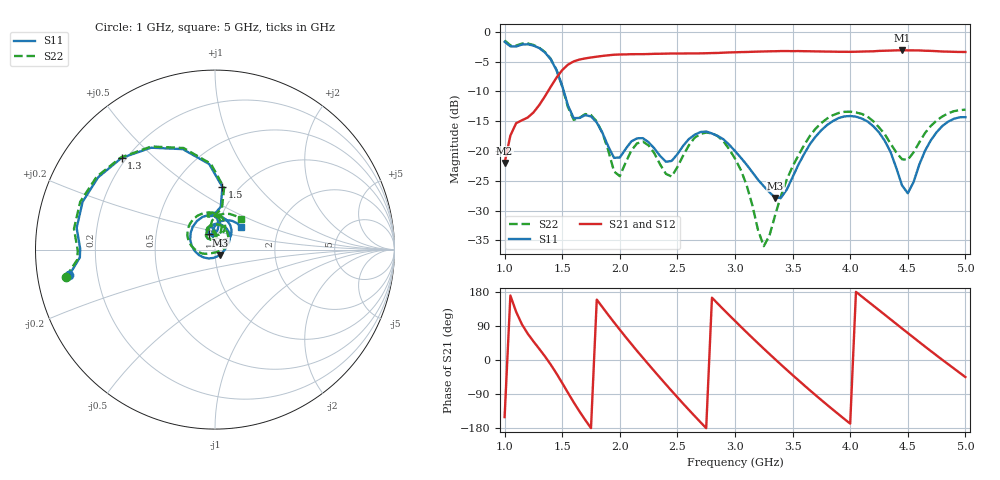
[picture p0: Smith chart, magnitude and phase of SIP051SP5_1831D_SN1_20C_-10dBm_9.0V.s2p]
# GHz  S  dB  R  50
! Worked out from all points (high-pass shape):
!   81 points, 1 GHz to 5 GHz, reference 50 ohm
!   highest |S21| = -3.12 dB at 4.45 GHz (marker M1); lowest = -22.0 dB at 1 GHz (marker M2)
!   |S21| within 3 dB of the highest: 1.518 GHz to end of sweep
!   lowest |S11| = -27.9 dB at 3.35 GHz (marker M3), VSWR 1.08, Z = 52.7 - j3.11 ohm
!   |S11| at or under -10 dB: 1.514 GHz to end of sweep
!   |S22| runs from -36.0 to -1.5 dB; largest |S21 - S12| = 0.002
!   S11 on the Smith chart (normalised r, x): 1 GHz: 0.10, -0.09; 1.3 GHz: 0.18, +0.40; 1.5 GHz: 0.84, +0.67; 2.5 GHz: 0.92, +0.16; 5 GHz: 1.29, +0.34
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1  -1.69 -170.2  -22.02 -150.6  -22.03 -150.5  -1.47 -169.7
1.1  -2.48 179.6  -15.35 127.2  -15.34 127.2  -2.33 -179.7
1.3  -2.74 135.6  -12.32 29.7  -12.35 29.6  -2.68 135.6
1.5  -9.10 83.2  -6.44 -60.7  -6.42 -60.8  -9.19 81.6
1.6  -14.50 93.5  -4.98 -111.8  -4.97 -111.8  -14.79 92.9
1.7  -14.01 100.4  -4.48 -158.3  -4.49 -158.3  -13.81 100.6
1.85  -17.00 81.3  -4.06 139.0  -4.05 139.0  -17.02 73.8
2  -21.11 109.3  -3.82 79.9  -3.82 80.0  -24.23 110.7
2.2  -17.86 99.9  -3.77 6.0  -3.77 5.9  -18.44 103.2
2.35  -20.85 90.9  -3.70 -47.0  -3.71 -47.0  -22.27 87.5
2.5  -20.55 111.7  -3.66 -98.3  -3.66 -98.3  -22.70 123.6
2.75  -16.75 79.3  -3.62 -179.9  -3.62 -180.0  -16.92 89.1
3  -20.02 35.1  -3.45 103.1  -3.44 103.2  -21.30 32.3
3.25  -25.93 -7.7  -3.32 29.7  -3.31 29.8  -35.98 -72.2
3.35  -27.89 -46.9  -3.28 1.5  -3.28 1.6  -30.67 -136.2
3.55  -22.33 -144.7  -3.25 -53.2  -3.25 -53.4  -20.77 -171.2
3.7  -17.60 170.4  -3.31 -92.9  -3.30 -92.9  -16.26 162.5
4.05  -14.25 89.1  -3.36 179.8  -3.37 179.8  -13.55 98.7
4.35  -20.16 36.2  -3.17 107.4  -3.17 107.4  -18.77 63.8
4.45  -25.80 44.8  -3.12 83.2  -3.12 83.2  -21.40 75.2
4.75  -16.87 85.7  -3.26 12.0  -3.27 12.0  -14.90 90.3
5  -14.34 41.1  -3.40 -45.0  -3.41 -45.0  -13.09 50.1
